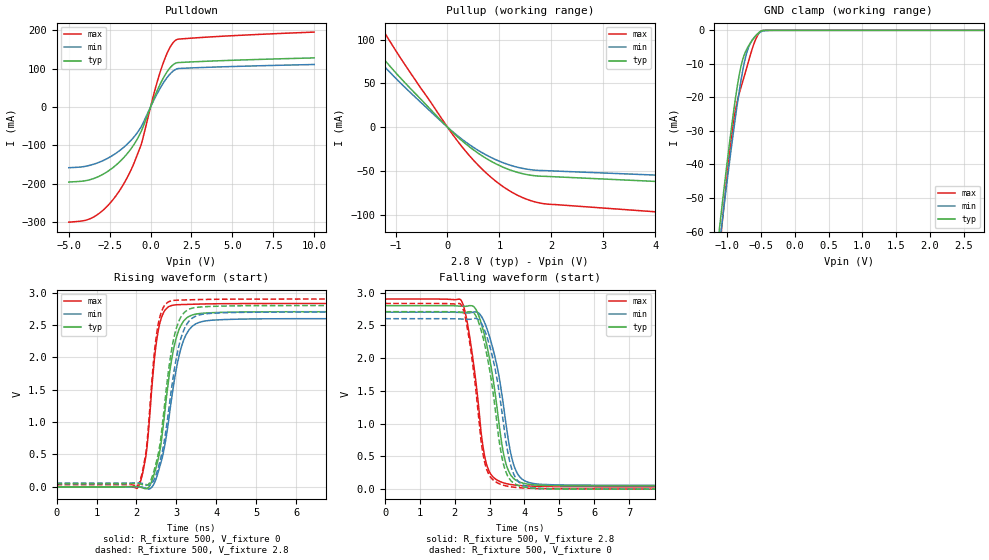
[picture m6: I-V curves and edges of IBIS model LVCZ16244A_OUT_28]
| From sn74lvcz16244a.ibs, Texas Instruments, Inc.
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[Model]   LVCZ16244A_OUT_28
Model_type  3-state
Enable   Active-Low
Vref =   0
Rref =   500
Cref =   50p
Vmeas =   1.5
| variable   typ   min   max
C_comp   6.74pF   5.83pF   7.84pF
| C_pullup   7.97pF   7.27pF   8.69pF
| C_pulldown   11.22pF   6.80pF   16.87pF
| C_tri-state   6.74pF   5.83pF   7.84pF
[Temperature Range]   40   100   -40
| Ambient temperature   25   85   -40
[Voltage range]   2.8   2.7   2.9
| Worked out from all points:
|   slope of the pulldown table from 0 to 0.42 V, typ, clamps not added: 9.52 ohm
|   slope of the pullup table from 0 to 0.42 V, typ, clamps not added: 18.9 ohm
|   GND clamp passes 1 mA (typ) near -0.55 V on its own axis
|   rising waveform, R_fixture 500, V_fixture 0: 20-80 % time 360ps typ, 417ps min, 252ps max; typ from 0 V to 2.71 V
|   falling waveform, R_fixture 500, V_fixture 2.8: 20-80 % time 483ps typ, 512ps min, 396ps max; typ from 2.8 V to 0.049 V
|   rising waveform, R_fixture 500, V_fixture 2.8: 20-80 % time 348ps typ, 398ps min, 245ps max; typ from 0.049 V to 2.8 V
|   falling waveform, R_fixture 500, V_fixture 0: 20-80 % time 459ps typ, 485ps min, 382ps max; typ from 2.71 V to 0 V
[GND Clamp]
| LVCZ16244A_OUT_28
|   Voltage   I(typ)   I(min)   I(max)
-5V       -857.7mA   -821.7mA   -988.1mA
-1.11V    -57.84mA   -62.7mA    -64.27mA
-1.08V    -52.56mA   -57.62mA   -58.21mA
-970mV    -33.97mA   -39.61mA   -37.24mA
-915mV    -25.37mA   -31.09mA   -28.29mA
-865mV    -18.28mA   -23.77mA   -22.25mA
-800mV    -10.93mA   -15.21mA   -17.15mA
-740mV    -6.841mA   -8.889mA   -13.03mA
-685mV    -4.623mA   -5.06mA    -9.179mA
-595mV    -1.988mA   -1.988mA   -3.41mA
-505mV    -261.8uA   -480.2uA   -291.5uA
2.8V      10.54pA    5.139nA    5.565pA
[Pulldown]
| LVCZ16244A_OUT_28
|   Voltage   I(typ)   I(min)   I(max)
-5V       -196.1mA   -158.7mA   -301mA
-3.965V   -192.5mA   -154.8mA   -295.8mA
-3.23V    -182.7mA   -145.9mA   -280.6mA
-2.42V    -162.3mA   -129.1mA   -248.4mA
-1.645V   -132.5mA   -105.5mA   -201.1mA
-1.11V    -104mA     -83.1mA    -156.5mA
-575mV    -63.9mA    -51.55mA   -98.17mA
260mV     28.17mA    22.97mA    43.38mA
770mV     74.8mA     61.94mA    114.5mA
1.16V     100.6mA    84.64mA    153.5mA
1.515V    114mA      97.66mA    173.8mA
10V       128.1mA    110.9mA    195.6mA
[Pullup]
| LVCZ16244A_OUT_28
|   Voltage   I(typ)   I(min)   I(max)
-5V       333.4mA    296.8mA    465.5mA
-2.005V   131.4mA    116.7mA    185.4mA
-1.78V    116.1mA    103.2mA    164mA
-1.3V     82.84mA    74.22mA    116.3mA
10mV      -612.7uA   -545.6uA   -877uA
445mV     -23.44mA   -20.87mA   -34.02mA
730mV     -35.11mA   -31.24mA   -51.45mA
1.065V    -45.54mA   -40.46mA   -67.62mA
1.365V    -51.87mA   -46mA      -78.16mA
1.715V    -55.66mA   -49.23mA   -85.74mA
7.61V     -71.67mA   -63.26mA   -112mA
10V       -78.15mA   -68.94mA   -122mA
[Ramp]
| LVCZ16244A_OUT_28
| variable   typ   min   max
dV/dt_r   1.64/3.68E-10   1.58/4.31E-10   1.71/2.56E-10
dV/dt_f   1.65/4.90E-10   1.59/5.20E-10   1.72/4.01E-10
R_load = 500
[Rising Waveform]
| LVCZ16244A_OUT_28
R_fixture =   500
C_fixture =   0
L_fixture =   0
V_fixture =   0
V_fixture_min = 0
V_fixture_max = 0
|   Time   V(typ)   V(min)   V(max)
0s        74.8pV     2.779nV    47.08pV
2.04ns    2.998mV    5.389mV    -3.485mV
2.24ns    -25.99mV   -21.31mV   494.1mV
2.435ns   183.9mV    43.74mV    1.892V
2.55ns    450.5mV    243.9mV    2.432V
2.715ns   1.193V     667.4mV    2.73V
2.91ns    2.071V     1.498V     2.805V
3.265ns   2.613V     2.377V     2.817V
3.89ns    2.689V     2.574V     2.827V
24.99ns   2.705V     2.598V     2.831V
[Falling Waveform]
| LVCZ16244A_OUT_28
R_fixture =   500
C_fixture =   0
L_fixture =   0
V_fixture =   2.8
V_fixture_min = 2.7
V_fixture_max = 2.9
|   Time   V(typ)   V(min)   V(max)
0s        2.8V       2.7V       2.9V
2.155ns   2.792V     2.696V     2.896V
2.335ns   2.791V     2.69V      2.605V
2.575ns   2.766V     2.705V     1.764V
2.91ns    2.214V     2.466V     380mV
3.245ns   1.094V     1.788V     130.1mV
3.515ns   312.1mV    826.8mV    80.52mV
3.82ns    117.4mV    218.2mV    57.8mV
4.47ns    58.58mV    73.86mV    42.86mV
24.99ns   48.99mV    57.97mV    32.97mV
[Rising Waveform]
| LVCZ16244A_OUT_28
R_fixture =   500
C_fixture =   0
L_fixture =   0
V_fixture =   2.8
V_fixture_min = 2.7
V_fixture_max = 2.9
|   Time   V(typ)   V(min)   V(max)
0s        48.82mV    57.91mV    32.85mV
2.04ns    51.57mV    63.13mV    30.29mV
2.24ns    23.32mV    36.42mV    550.4mV
2.435ns   242.4mV    105.3mV    2.002V
2.54ns    500.1mV    291.4mV    2.502V
2.69ns    1.197V     688.3mV    2.791V
2.9ns     2.192V     1.621V     2.877V
3.22ns    2.707V     2.47V      2.887V
3.81ns    2.785V     2.677V     2.895V
24.99ns   2.8V       2.7V       2.9V
[Falling Waveform]
| LVCZ16244A_OUT_28
R_fixture =   500
C_fixture =   0
L_fixture =   0
V_fixture =   0
V_fixture_min = 0
V_fixture_max = 0
|   Time   V(typ)   V(min)   V(max)
0s        2.708V     2.601V     2.833V
2.155ns   2.701V     2.596V     2.829V
2.335ns   2.7V       2.591V     2.527V
2.57ns    2.672V     2.605V     1.665V
2.895ns   2.114V     2.367V     330.6mV
3.185ns   1.109V     1.755V     107.4mV
3.5ns     219.7mV    625mV      45.99mV
3.8ns     60.63mV    130.7mV    24.13mV
4.44ns    7.862mV    12.21mV    9.738mV
24.99ns   168.7uV    55.24uV    120.7uV
